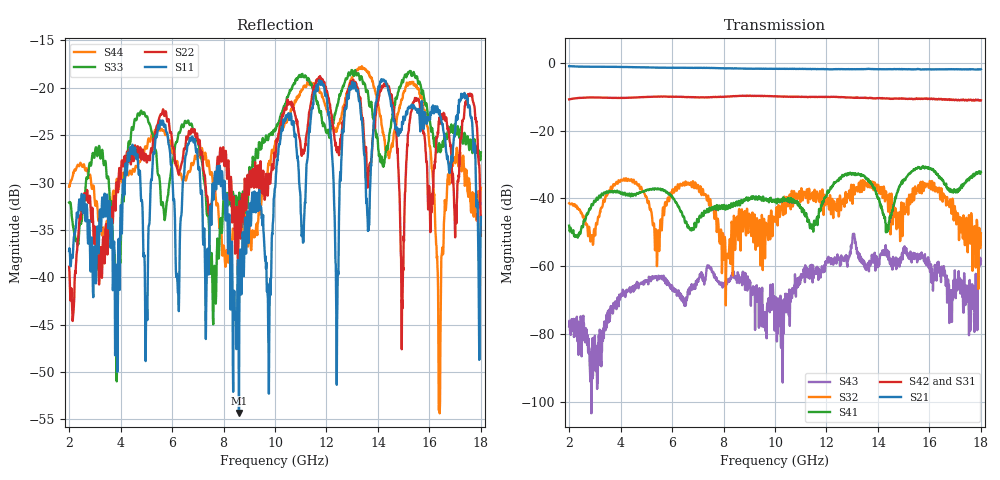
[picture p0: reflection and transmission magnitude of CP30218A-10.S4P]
! Amtery
! Email: info@amtery.com
! Phone: 886-2-2883-7839
! Model Number: CP30218A-10
! 4-port S-parameter measurement data for Dual-Directional Coupler
! Frequency Range: 0.5 GHz to 18 GHz
! Port 1: Input
! Port 2: Output
! Port 3: Coupled Forward
! Port 4: Coupled Reverse
# Hz S dB R 50
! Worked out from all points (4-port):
!   1281 points, 2 GHz to 18 GHz, reference 50 ohm
!   strongest paths, dB at 2 GHz, 6 GHz, 10 GHz, 14 GHz, 18 GHz:
!     S21: -1.0, -1.5, -1.8, -1.9, -1.9
!     S42: -10.8, -10.0, -9.9, -10.4, -11.1
!     S31: -10.8, -10.1, -10.0, -10.4, -11.0
!     S41: -48.1, -39.4, -40.9, -39.8, -32.2
!     S32: -41.5, -38.1, -45.8, -36.0, -50.3
!     S43: -77.8, -65.7, -70.4, -59.5, -58.6
!   lowest |S11| = -54.3 dB at 8.6 GHz (marker M1), VSWR 1.00, Z = 49.8 + j0.0779 ohm
!   |S11| at or under -10 dB: start of sweep to end of sweep
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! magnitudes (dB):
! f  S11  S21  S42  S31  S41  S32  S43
! 2 GHz  -37.2  -1.0  -10.8  -10.8  -48.1  -41.5  -77.8
! 8.6 GHz  -54.3  -1.7  -9.8  -9.8  -40.7  -43.4  -63.4
! 11.75 GHz  -19.4  -1.9  -10.1  -10.1  -43.2  -37.9  -61.3
! 12.4 GHz  -51.3  -1.9  -10.1  -10.2  -35.0  -43.8  -58.8
! 13.05 GHz  -19.9  -1.9  -10.3  -10.3  -32.7  -36.0  -50.8
! 16.38 GHz  -22.8  -1.9  -10.7  -10.8  -34.0  -36.9  -60.1
! 18 GHz  -33.6  -1.9  -11.1  -11.0  -32.2  -50.3  -58.6
